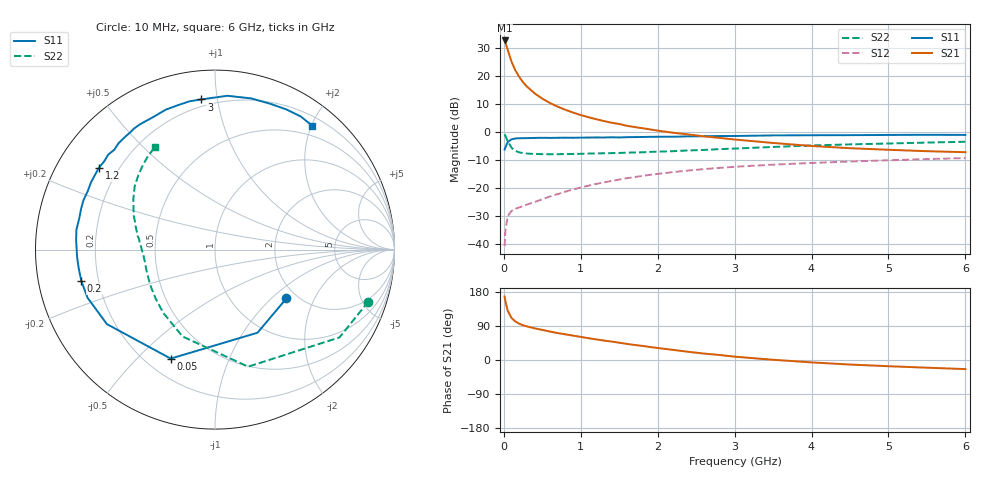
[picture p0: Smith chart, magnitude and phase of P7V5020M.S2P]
! SIEMENS Small Signal Semiconductors
! BFP196
! Si NPN RF Bipolar Junction Transistor in SOT143
! VCE = 0.5 V  IC = 20 mA
! Common Emitter S-Parameters:  May  1996
# GHz  S  MA  R  50
!  f  S11  S21  S12  S22
! GHz  MAG  ANG  MAG  ANG  MAG  ANG  MAG  ANG
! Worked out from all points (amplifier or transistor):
!   36 points, 10 MHz to 6 GHz, reference 50 ohm
!   highest |S21| = 32.6 dB at 10 MHz (marker M1)
!   |S21| within 3 dB of that: start of sweep to 46.06 MHz
!   unconditionally stable (mu >= 1): 572.6 MHz to end of sweep
!   at 250 MHz: K = 0.64, MSG = 22.1 dB, |S12| = -26.6 dB
!   at 1.4 GHz: K = 1.14, MAG = 8.1 dB, |S12| = -17.6 dB
!   at 6 GHz: K = 1.05, MAG = -0.3 dB, |S12| = -9.4 dB
!   S11 on the Smith chart (normalised r, x): 10 MHz: 1.76, -1.25; 50 MHz: 0.30, -0.63; 200 MHz: 0.13, -0.11; 1.2 GHz: 0.13, +0.31; 3 GHz: 0.16, +0.90; 6 GHz: 0.34, +2.01
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0.01  0.482 -34.3  42.88 167.5  0.009 78.9  0.9023 -18.7
0.02  0.5202 -62.9  39.65 154.8  0.0168 67.6  0.8488 -35.2
0.05  0.6554 -112.1  29.15 130.2  0.0309 46.9  0.6779 -74.2
0.1  0.7314 -145.4  17.86 110.9  0.0385 34.6  0.5167 -110.5
0.15  0.7591 -159.3  12.5 101.6  0.0418 32.9  0.4554 -129.2
0.2  0.7651 -166.9  9.571 95.7  0.0444 33.4  0.428 -140.7
0.25  0.7667 -172.7  7.66 91.7  0.047 35.2  0.4145 -148.6
0.3  0.7694 -176.9  6.427 88.6  0.0498 37.5  0.4074 -153.7
0.4  0.7755 176.1  4.869 83.5  0.0556 41.1  0.4001 -161.0
0.5  0.7801 171.9  3.904 79.4  0.0621 44.0  0.3976 -165.8
0.6  0.7761 167.2  3.263 75.1  0.0697 46.5  0.3962 -169.1
0.7  0.78 162.9  2.811 71.0  0.0768 47.5  0.3972 -171.8
0.9  0.7802 155.4  2.202 64.3  0.093 48.8  0.3999 -176.0
1.1  0.7874 148.3  1.819 57.5  0.1086 49.0  0.4069 -179.1
1.2  0.7915 144.8  1.676 54.4  0.1165 48.8  0.4093 179.3
1.6  0.8001 132.2  1.279 42.5  0.1477 45.2  0.4225 174.2
2.2  0.8147 115.1  0.96 26.7  0.1901 38.0  0.4496 166.3
3  0.8401 95.2  0.727 8.8  0.2363 27.1  0.5003 155.0
3.5  0.8598 85.4  0.63 0.6  0.2581 20.6  0.5349 148.3
4.5  0.8691 69.1  0.508 -12.0  0.2937 8.8  0.5946 136.0
5.5  0.8823 57.2  0.449 -20.3  0.3247 -1.6  0.6407 125.7
6  0.8773 51.9  0.431 -24.0  0.3385 -7.3  0.6617 120.4
